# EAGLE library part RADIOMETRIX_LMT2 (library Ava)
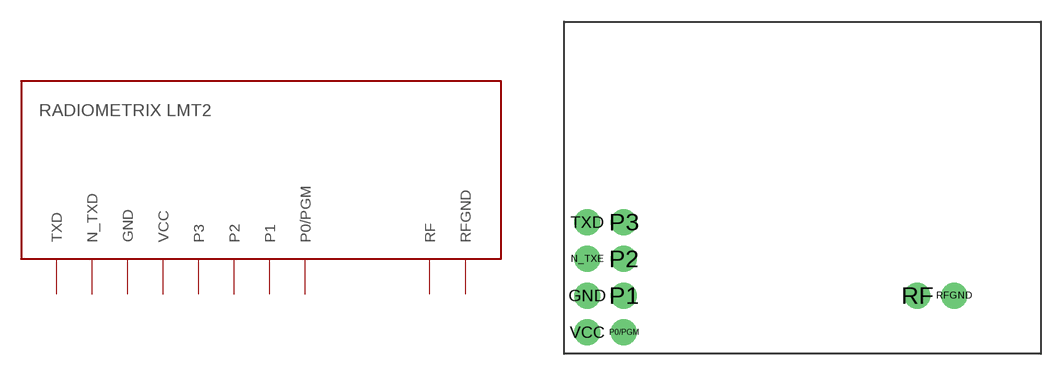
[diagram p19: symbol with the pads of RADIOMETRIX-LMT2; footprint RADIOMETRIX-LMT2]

Designator prefix -

## RADIOMETRIX_LMT2  [RADIOMETRIX-LMT2]
GND  GND  pwr
N_TXE  N_TXD
P0/PGM  P0/PGM
P1  P1
P2  P2
P3  P3
RF  RF
RFGND  RFGND
TXD  TXD
VCC  VCC  pwr

## Footprint RADIOMETRIX-LMT2 (pad centres in mm)
drill 1.2: GND -14.91,-7.39; N_TXE -14.91,-4.85; P0/PGM -12.37,-9.93; P1 -12.37,-7.39; P2 -12.37,-4.85; P3 -12.37,-2.31; RF 7.95,-7.39; RFGND 10.49,-7.39; TXD -14.91,-2.31; VCC -14.91,-9.93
